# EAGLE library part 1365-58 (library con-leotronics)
DUAL ROW STRAIGHT HEADER 1364 SERIES. 1.27mm x 1.27mm. Without Fixing Post. SMT Source: http://www.leotronics.co.uk/Conexcon/Data%20Sheets/sec.%20A/1364ing.pdf
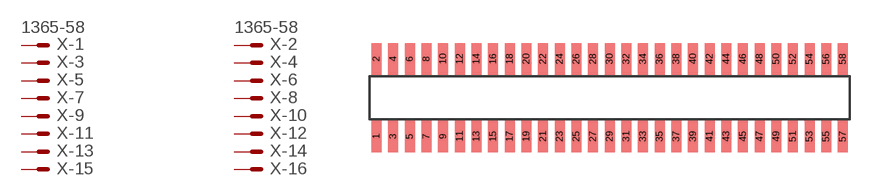
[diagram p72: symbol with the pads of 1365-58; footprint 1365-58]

Designator prefix X; gates -1=MVAL -2=MVAL -3=M -4=M -5=M -6=M -7=M -8=M -9=M -10=M -11=M -12=M -13=M -14=M -15=M -16=M -17=M -18=M -19=M -20=M -21=M -22=M -23=M -24=M -25=M -26=M -27=M -28=M -29=M -30=M -31=M -32=M -33=M -34=M -35=M -36=M -37=M -38=M -39=M -40=M -41=M -42=M -43=M -44=M -45=M -46=M -47=M -48=M -49=M -50=M -51=M -52=M -53=M -54=M -55=M -56=M -57=M -58=M

## 1365-58 (OC_FARNELL: unknown; OC_NEWARK: unknown)  [1365-58]
1  -1:S  pas
2  -2:S  pas
3  -3:S  pas
4  -4:S  pas
5  -5:S  pas
6  -6:S  pas
7  -7:S  pas
8  -8:S  pas
9  -9:S  pas
10  -10:S  pas
11  -11:S  pas
12  -12:S  pas
13  -13:S  pas
14  -14:S  pas
15  -15:S  pas
16  -16:S  pas
17  -17:S  pas
18  -18:S  pas
19  -19:S  pas
20  -20:S  pas
21  -21:S  pas
22  -22:S  pas
23  -23:S  pas
24  -24:S  pas
25  -25:S  pas
26  -26:S  pas
27  -27:S  pas
28  -28:S  pas
29  -29:S  pas
30  -30:S  pas
31  -31:S  pas
32  -32:S  pas
33  -33:S  pas
34  -34:S  pas
35  -35:S  pas
36  -36:S  pas
37  -37:S  pas
38  -38:S  pas
39  -39:S  pas
40  -40:S  pas
41  -41:S  pas
42  -42:S  pas
43  -43:S  pas
44  -44:S  pas
45  -45:S  pas
46  -46:S  pas
47  -47:S  pas
48  -48:S  pas
49  -49:S  pas
50  -50:S  pas
51  -51:S  pas
52  -52:S  pas
53  -53:S  pas
54  -54:S  pas
55  -55:S  pas
56  -56:S  pas
57  -57:S  pas
58  -58:S  pas

## Footprint 1365-58 (pad centres in mm)
DUAL ROW STRAIGHT HEADER 1364 SERIES. 1.27mm x 1.27mm. Without Fixing Post. SMT Source: http://www.leotronics.co.uk/Conexcon/Data%20Sheets/sec.%20A/1364ing.pdf
smd 0.76 x 2.4: 1 -17.78,-2.95; 2 -17.78,2.95; 3 -16.51,-2.95; 4 -16.51,2.95; 5 -15.24,-2.95; 6 -15.24,2.95; 7 -13.97,-2.95; 8 -13.97,2.95; 9 -12.7,-2.95; 10 -12.7,2.95; 11 -11.43,-2.95; 12 -11.43,2.95; 13 -10.16,-2.95; 14 -10.16,2.95; 15 -8.89,-2.95; 16 -8.89,2.95; 17 -7.62,-2.95; 18 -7.62,2.95; 19 -6.35,-2.95; 20 -6.35,2.95; 21 -5.08,-2.95; 22 -5.08,2.95; 23 -3.81,-2.95; 24 -3.81,2.95; 25 -2.54,-2.95; 26 -2.54,2.95; 27 -1.27,-2.95; 28 -1.27,2.95; 29 0,-2.95; 30 0,2.95; 31 1.27,-2.95; 32 1.27,2.95; 33 2.54,-2.95; 34 2.54,2.95; 35 3.81,-2.95; 36 3.81,2.95; 37 5.08,-2.95; 38 5.08,2.95; 39 6.35,-2.95; 40 6.35,2.95; 41 7.62,-2.95; 42 7.62,2.95; 43 8.89,-2.95; 44 8.89,2.95; 45 10.16,-2.95; 46 10.16,2.95; 47 11.43,-2.95; 48 11.43,2.95; 49 12.7,-2.95; 50 12.7,2.95; 51 13.97,-2.95; 52 13.97,2.95; 53 15.24,-2.95; 54 15.24,2.95; 55 16.51,-2.95; 56 16.51,2.95; 57 17.78,-2.95; 58 17.78,2.95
